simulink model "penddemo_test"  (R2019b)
settings: Solver=ode4  StartTime=0  StopTime=20  FixedStep=0.02  MaxStep=0.02  RelTol=1e-3  AbsTol=1e-6
undefined symbols (not defined in the file or in its folder): Reference

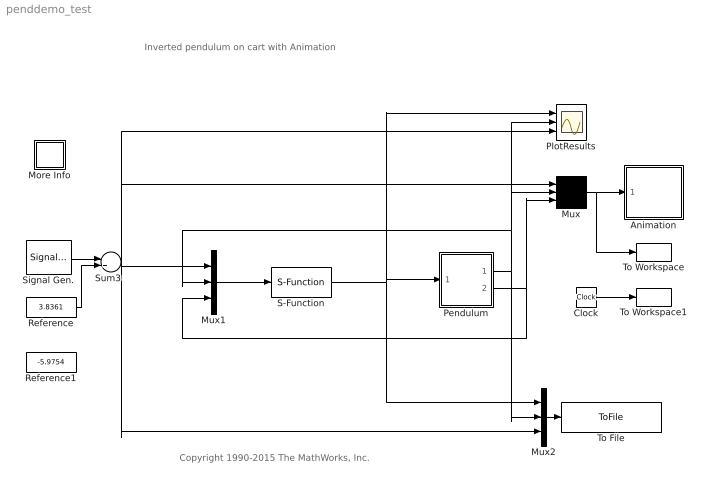
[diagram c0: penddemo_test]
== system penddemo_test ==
  note: Inverted pendulum on cart with Animation
  note: Copyright 1990-2015 The MathWorks, Inc.
  Animation : Subsystem  mask(Pendulum plot){RefBlock=Reference}
      mask prompts: RefBlock "DC reference signal block name:"
      mask help: Pendulum plot
  Clock : Clock
  More Info : Subsystem
  Mux : Mux  Inputs=3
  Mux1 : Mux  Inputs=3
  Mux2 : Mux  Inputs=3
  Pendulum : Subsystem  mask(Inverted pendulum on cart){Mcart=0.455, m=0.21, l=0.61/2, g=9.8}
      mask prompts: Mcart "Mass of cart (kg):"; m "Mass of pendulum (kg):"; l "Distance to pendulum center of mass(m):"; g "Acceleration of gravity (m/s^2):"
      mask help: Unmask and double-click to see dynamics
  PlotResults : Scope  NumInputPorts=3
  Reference : Constant  Value=3.8361
  Reference1 : Constant  Value=-5.9754
  S-Function : S-Function  FunctionName=modbusCom  SFunctionDeploymentMode=off  EnableBusSupport=off
  Signal Gen. : SignalGenerator  WaveForm=square  Amplitude=2  Frequency=1.5  Units=rad/sec
  Sum3 : Sum
  To File : ToFile  Commented=on  Filename=E:\MATLAB\simData\sim_penddemo.mat  MatrixName=log  SaveFormat=Timeseries
  To Workspace : ToWorkspace  VariableName=ytest  SampleTime=0.1
  To Workspace1 : ToWorkspace  VariableName=ttest  SampleTime=0.1
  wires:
  Mux/1 -> To Workspace/1, Animation/1(in_1)
  Pendulum/2(Pendulum) -> Mux/3, Mux1/3
  Sum3/1 -> Mux2/3, PlotResults/3, Mux/1, Mux1/1
  Reference/1 -> Sum3/2
  Signal Gen./1 -> Sum3/1
  Pendulum/1(Cart) -> Mux2/2, PlotResults/2, Mux/2, Mux1/2
  Clock/1 -> To Workspace1/1
  Mux1/1 -> S-Function/1
  S-Function/1 -> Mux2/1, Pendulum/1(U), PlotResults/1
  Mux2/1 -> To File/1

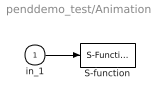
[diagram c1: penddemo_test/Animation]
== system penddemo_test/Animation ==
  in_1 : Inport
  S-function : S-Function  FunctionName=pendan  Parameters=RefBlock  SFunctionDeploymentMode=off  EnableBusSupport=off
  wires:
  in_1/1 -> S-function/1

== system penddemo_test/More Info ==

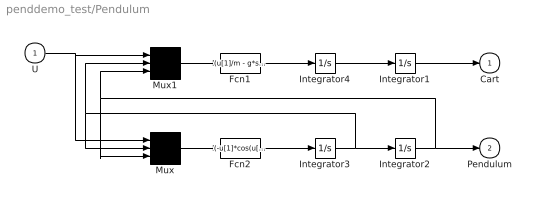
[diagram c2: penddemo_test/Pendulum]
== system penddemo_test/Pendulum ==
  U : Inport
  Fcn1 : Fcn  Expr=(u[1]/m - g*sin(u[3])*cos(u[3]) + l*power(u[2],2)*sin(u[3]))/(Mcart/m + power(sin(u[3]),2))
  Fcn2 : Fcn  Expr=(-u[1]*cos(u[3])/m + (Mcart+m)*g*sin(u[3])/m - l*power(u[2],2)*sin(u[3])*cos(u[3]))/(l*(Mcart/m + power(sin(u[3]),2)))
  Integrator{1..4} (4 alike) : Integrator
  Mux : Mux  Inputs=3
  Mux1 : Mux  Inputs=3
  Cart : Outport  InitialOutput=0  VectorParamsAs1DForOutWhenUnconnected=off
  Pendulum : Outport  Port=2  InitialOutput=0  VectorParamsAs1DForOutWhenUnconnected=off
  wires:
  Integrator1/1 -> Cart/1
  Fcn2/1 -> Integrator3/1
  Mux/1 -> Fcn2/1
  Mux1/1 -> Fcn1/1
  Fcn1/1 -> Integrator4/1
  Integrator4/1 -> Integrator1/1
  U/1 -> Mux1/1, Mux/1
  Integrator3/1 -> Integrator2/1, Mux1/2, Mux/2
  Integrator2/1 -> Pendulum/1, Mux1/3, Mux/3
